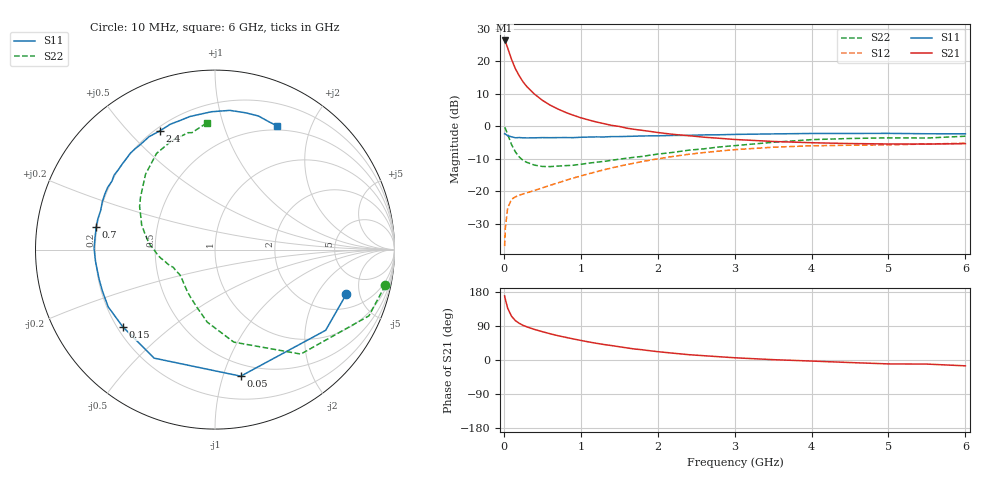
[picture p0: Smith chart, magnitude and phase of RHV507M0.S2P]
! SIEMENS Small Signal Semiconductors
! BFR106
! Si NPN RF Bipolar Junction Transistor in SOT23
! VCE = 0.5 V  IC = 7 mA
! Common Emitter S-Parameters:  August  1996
# GHz  S  MA  R  50
!  f  S11  S21  S12  S22
! GHz  MAG  ANG  MAG  ANG  MAG  ANG  MAG  ANG
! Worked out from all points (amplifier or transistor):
!   36 points, 10 MHz to 6 GHz, reference 50 ohm
!   highest |S21| = 26.5 dB at 10 MHz (marker M1)
!   |S21| within 3 dB of that: start of sweep to 59.51 MHz
!   unconditionally stable (mu >= 1): 502 MHz to end of sweep
!   at 250 MHz: K = 0.64, MSG = 17.2 dB, |S12| = -20.7 dB
!   at 1.4 GHz: K = 1.17, MAG = 4.0 dB, |S12| = -12.8 dB
!   at 6 GHz: K = 1.03, MAG = -1.1 dB, |S12| = -5.2 dB
!   S11 on the Smith chart (normalised r, x): 10 MHz: 3.02, -3.72; 50 MHz: 0.39, -1.15; 150 MHz: 0.22, -0.35; 700 MHz: 0.20, +0.09; 2.4 GHz: 0.22, +0.62; 6 GHz: 0.45, +1.53
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0.01  0.7727 -18.7  21.05 169.1  0.0144 82.3  0.9691 -11.9
0.02  0.7631 -36.1  20.33 159.9  0.0277 72.8  0.9336 -23.3
0.05  0.7197 -78.5  16.08 136.5  0.0559 53.3  0.7533 -50.6
0.1  0.6934 -119.3  10.77 115.5  0.0755 38.7  0.5261 -78.5
0.15  0.6701 -140.0  7.734 103.9  0.0827 33.4  0.4069 -96.0
0.2  0.6752 -151.8  6.014 96.9  0.0874 32.4  0.3393 -106.9
0.25  0.6683 -159.8  4.852 91.4  0.0918 32.7  0.3002 -116.6
0.3  0.6663 -165.7  4.091 87.4  0.0954 34.2  0.2802 -123.4
0.4  0.6692 -174.5  3.132 80.6  0.1038 37.0  0.2541 -133.9
0.5  0.6739 179.3  2.531 74.8  0.1136 39.8  0.2426 -140.9
0.6  0.6717 173.5  2.134 69.3  0.1241 42.2  0.2411 -145.6
0.7  0.674 169.0  1.862 64.3  0.1352 44.5  0.2456 -150.1
0.9  0.6732 161.0  1.492 55.7  0.1606 47.1  0.2529 -157.2
1.1  0.6873 153.2  1.262 47.8  0.1869 48.2  0.2726 -162.2
1.3  0.6893 146.4  1.105 40.9  0.2154 48.0  0.2899 -167.9
1.6  0.7033 137.1  0.941 31.9  0.2589 46.5  0.3253 -176.0
2.2  0.7285 120.3  0.756 18.0  0.3459 39.4  0.3995 167.4
2.4  0.7297 114.7  0.722 14.1  0.373 36.3  0.4312 161.4
3.5  0.7683 91.5  0.588 0.9  0.4798 18.3  0.5709 132.7
4.5  0.781 77.4  0.546 -6.7  0.5145 3.7  0.6533 111.5
5.5  0.7726 67.0  0.536 -10.8  0.5374 -4.8  0.6639 101.2
6  0.7718 63.3  0.544 -15.4  0.5523 -11.1  0.708 93.6
